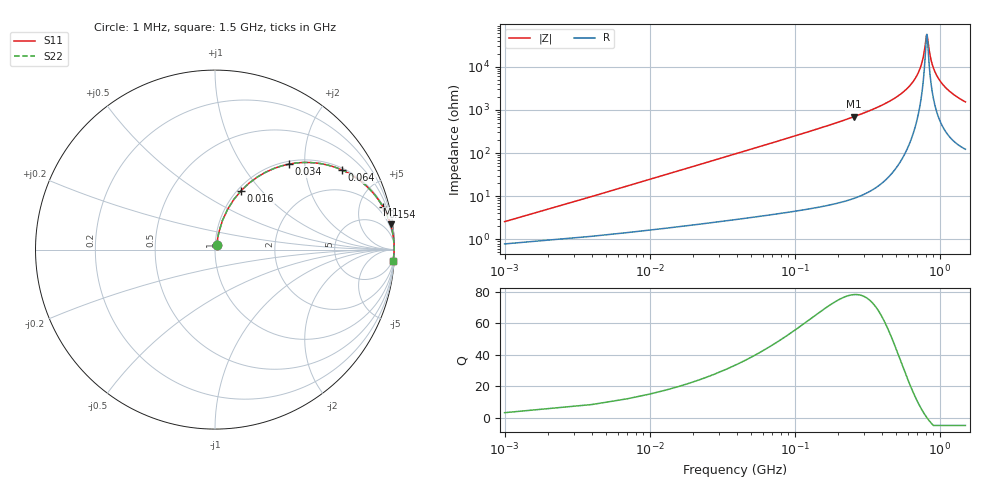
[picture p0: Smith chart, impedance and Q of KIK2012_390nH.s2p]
!version-2
!date-01.2022
!Series
# MHz S RI R 50
!Freq ReS11 ImS11 ReS21 ImS21 ReS12 ImS12 ReS22 ImS22
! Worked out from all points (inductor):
!   501 points, 1 MHz to 1.5 GHz, reference 50 ohm
!   read as one part in series: L = 390 nH near 7 MHz
!   highest Q = 78.2 at 256 MHz (marker M1), where L = 433 nH
!   self-resonance near 811 MHz
!   S11 on the Smith chart (normalised r, x): 1 MHz: 1.02, +0.05; 16 MHz: 1.04, +0.78; 34 MHz: 1.05, +1.67; 64 MHz: 1.07, +3.16; 154 MHz: 1.11, +7.83; 1.5 GHz: 3, -31
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1  0.00836 0.0241  0.9916 -0.0241  0.9916 -0.0241  0.00836 0.0241
10  0.0702 0.2242  0.9298 -0.2242  0.9298 -0.2242  0.0702 0.2242
16  0.1457 0.3286  0.8543 -0.3286  0.8543 -0.3286  0.1457 0.3286
34  0.4136 0.4766  0.5864 -0.4766  0.5864 -0.4766  0.4136 0.4766
64  0.7093 0.4429  0.2907 -0.4429  0.2907 -0.4429  0.7093 0.4429
100  0.8565 0.3417  0.1435 -0.3417  0.1435 -0.3417  0.8565 0.3417
154  0.9357 0.2381  0.0643 -0.2381  0.0643 -0.2381  0.9357 0.2381
253  0.9775 0.1421  0.0225 -0.1421  0.0225 -0.1421  0.9775 0.1421
256  0.9781 0.1402  0.0219 -0.1402  0.0219 -0.1402  0.9781 0.1402
502  0.9963 0.0501  0.00368 -0.0501  0.00368 -0.0501  0.9963 0.0501
661  0.9982 0.0209  0.00182 -0.0209  0.00182 -0.0209  0.9982 0.0209
712  0.9983 0.0134  0.00167 -0.0134  0.00167 -0.0134  0.9983 0.0134
751  0.9983 0.00802  0.00166 -0.00802  0.00166 -0.00802  0.9983 0.00802
775  0.9983 0.00487  0.00169 -0.00487  0.00169 -0.00487  0.9983 0.00487
805  0.9982 0.00107  0.00175 -0.00107  0.00175 -0.00107  0.9982 0.00107
814  0.9982 -3.68e-05  0.00178 3.68e-05  0.00178 3.68e-05  0.9982 -3.68e-05
853  0.9981 -0.00471  0.00193 0.00471  0.00193 0.00471  0.9981 -0.00471
886  0.9979 -0.0085  0.0021 0.0085  0.0021 0.0085  0.9979 -0.0085
937  0.9976 -0.0141  0.00241 0.0141  0.00241 0.0141  0.9976 -0.0141
1003  0.9971 -0.021  0.00292 0.021  0.00292 0.021  0.9971 -0.021
1252  0.9944 -0.0441  0.00564 0.0441  0.00564 0.0441  0.9944 -0.0441
1500  0.9907 -0.0641  0.00934 0.0641  0.00934 0.0641  0.9907 -0.0641
